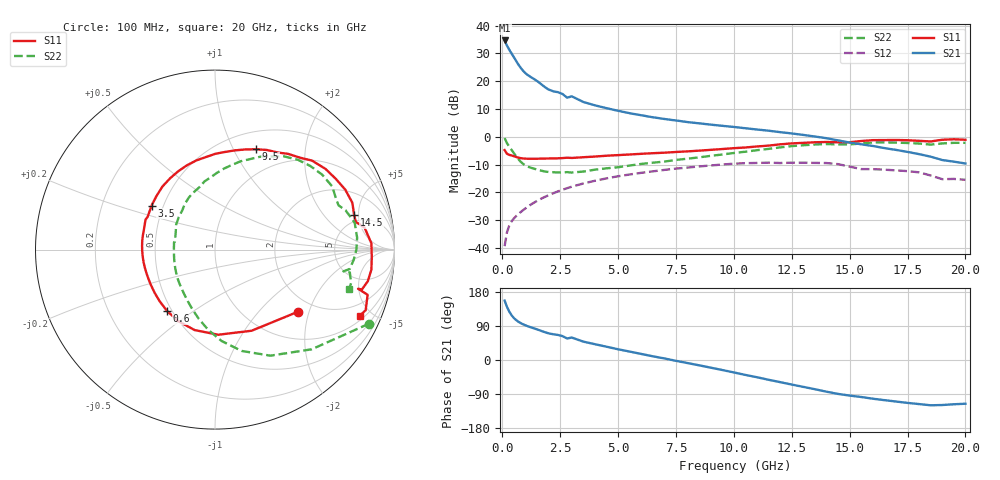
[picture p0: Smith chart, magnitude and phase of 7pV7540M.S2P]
! Infineon Technologies  Discrete & RF Semiconductors
! bfp620
! VCE = 0.75 V,  IC =  40 mA
! Common Emitter S-Parameters:  Sep 2002
# GHz  S  MA  R  50
!  f  S11  S21  S12  S22
! GHz  MAG  ANG  MAG  ANG  MAG  ANG  MAG  ANG
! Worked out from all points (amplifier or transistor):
!   59 points, 100 MHz to 20 GHz, reference 50 ohm
!   highest |S21| = 34.7 dB at 100 MHz (marker M1)
!   |S21| within 3 dB of that: start of sweep to 279.2 MHz
!   unconditionally stable (mu >= 1): 2.687 GHz to 2.911 GHz; 3.206 GHz to 10.21 GHz; 17.04 GHz to end of sweep
!   at 1 GHz: K = 0.84, MSG = 24.3 dB, |S12| = -25.7 dB
!   at 5.5 GHz: K = 1.04, MAG = 9.8 dB, |S12| = -13.5 dB
!   at 20 GHz: K = 1.46, MAG = -1.1 dB, |S12| = -15.4 dB
!   S11 on the Smith chart (normalised r, x): 100 MHz: 1.63, -1.70; 600 MHz: 0.47, -0.40; 3.5 GHz: 0.43, +0.26; 9.5 GHz: 0.70, +1.23; 14.5 GHz: 4.12, +4.39; 20 GHz: 1.23, -4.25
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0.1  0.5783 -36.7  54.21 156.8  0.0108 77.6  0.9521 -25.7
0.2  0.496 -65.7  43.88 140.6  0.0191 65.4  0.7737 -45.9
0.3  0.4747 -87.8  37.05 127.8  0.0253 61.0  0.6668 -62.4
0.4  0.4626 -104.1  31.67 118.1  0.0301 58.6  0.5836 -75.3
0.5  0.4485 -117.0  27.07 110.8  0.0341 57.2  0.5104 -85.9
0.6  0.434 -127.8  23.13 105.2  0.0376 56.5  0.4469 -95.1
0.7  0.422 -136.9  19.88 100.8  0.0411 56.1  0.3948 -103.4
0.8  0.4134 -144.5  17.32 97.2  0.0446 56.0  0.3549 -110.9
1  0.4053 -155.7  13.98 91.5  0.0517 56.1  0.3059 -123.3
1.3  0.4037 -166.7  11.44 84.9  0.0629 55.8  0.273 -136.7
1.8  0.4065 177.8  8.092 74.2  0.0816 53.5  0.2401 -159.0
2.8  0.4216 156.6  5.062 56.8  0.1192 45.9  0.2319 169.8
3  0.4173 154.2  5.36 59.2  0.1269 44.2  0.2279 169.0
3.5  0.43 145.2  4.237 48.5  0.145 39.3  0.2376 157.2
5  0.4695 122.2  2.942 28.3  0.1955 24.2  0.2839 130.1
7  0.5188 95.3  2.097 4.1  0.2543 3.7  0.3589 103.9
9.5  0.6034 67.9  1.58 -26.4  0.3177 -23.7  0.4816 78.6
10.5  0.6438 57.2  1.429 -39.4  0.3362 -36.5  0.5402 68.9
13.5  0.799 24.7  1.015 -77.1  0.3399 -72.1  0.7285 35.0
14.5  0.7987 14.0  0.864 -89.5  0.3229 -87.3  0.7319 23.1
17  0.8784 -7.3  0.583 -109.6  0.2496 -103.0  0.7878 0.0
20  0.8868 -24.6  0.332 -115.4  0.169 -113.8  0.7803 -16.3
